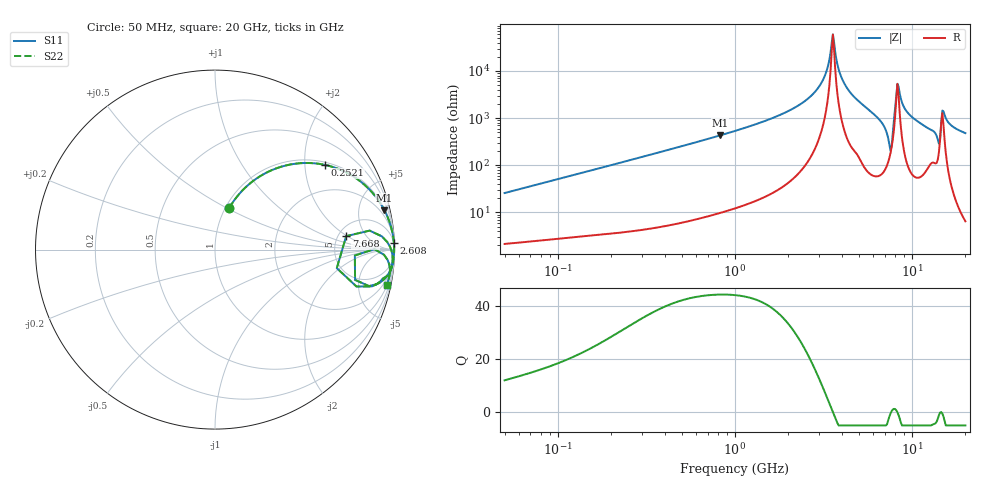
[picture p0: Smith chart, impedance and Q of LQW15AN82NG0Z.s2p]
!Murata Part Number: LQW15AN82NG0Z
!These Parameters are Measured in Series Mode Connection
!  o--[Z]--o
!Port1  Port2
!  o-------o
!Freq. Start=50[MHz] Stop=20[GHz], 401[Steps]
# Hz S RI R 50
!Freq.(Hz) S11(Real) S11(Imag) S21(Real) S21(Imag) S12(Real) S12(Imag) S22(Real) S22(Imag)
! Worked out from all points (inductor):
!   401 points, 50 MHz to 20 GHz, reference 50 ohm
!   read as one part in series: L = 81.5 nH near 51.52 MHz
!   highest Q = 44.2 at 823.1 MHz (marker M1), where L = 83.2 nH
!   self-resonance near 3.572 GHz
!   S11 on the Smith chart (normalised r, x): 50 MHz: 1.04, +0.51; 252.1 MHz: 1.08, +2.54; 2.608 GHz: 4, +53; 7.668 GHz: 5.90, +1.92; 20 GHz: 1.13, -9.63
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5e7  0.0794 0.2318  0.9206 -0.2318  0.9206 -0.2318  0.0794 0.2318
1.364002e8  0.3298 0.4482  0.6702 -0.4482  0.6702 -0.4482  0.3298 0.4482
2.520729e8  0.6138 0.4717  0.3862 -0.4717  0.3862 -0.4717  0.6138 0.4717
3.721004e8  0.7734 0.4059  0.2266 -0.4059  0.2266 -0.4059  0.7734 0.4059
8.230629e8  0.9443 0.2183  0.0557 -0.2183  0.0557 -0.2183  0.9443 0.2183
1e9  0.9625 0.1789  0.0375 -0.1789  0.0375 -0.1789  0.9625 0.1789
1.820564e9  0.9908 0.0825  0.00917 -0.0825  0.00917 -0.0825  0.9908 0.0825
2.608132e9  0.9968 0.0371  0.00317 -0.0371  0.00317 -0.0371  0.9968 0.0371
2.728004e9  0.9972 0.0318  0.00276 -0.0318  0.00276 -0.0318  0.9972 0.0318
3.216634e9  0.9982 0.0124  0.00182 -0.0124  0.00182 -0.0124  0.9982 0.0124
3.572216e9  0.9983 2.62e-05  0.00168 -2.62e-05  0.00168 -2.62e-05  0.9983 2.62e-05
3.908127e9  0.9981 -0.0109  0.00187 0.0109  0.00187 0.0109  0.9981 -0.0109
4.212059e9  0.9977 -0.0203  0.00232 0.0203  0.00232 0.0203  0.9977 -0.0203
6.601595e9  0.9801 -0.1092  0.0199 0.1092  0.0199 0.1092  0.9801 -0.1092
7.442007e9  0.7885 -0.2057  0.2115 0.2057  0.2115 0.2057  0.7885 -0.2057
7.668323e9  0.7311 0.075  0.2689 -0.075  0.2689 -0.075  0.7311 0.075
8.141811e9  0.9743 0.0174  0.0257 -0.0174  0.0257 -0.0174  0.9743 0.0174
8.389408e9  0.9857 -0.0156  0.0143 0.0156  0.0143 0.0156  0.9857 -0.0156
9.600142e9  0.9878 -0.0804  0.0122 0.0804  0.0122 0.0804  0.9878 -0.0804
1.396067e10  0.8582 -0.2035  0.1418 0.2035  0.1418 0.2035  0.8582 -0.2035
1.504638e10  0.9617 -0.0576  0.0383 0.0576  0.0383 0.0576  0.9617 -0.0576
2e10  0.9562 -0.198  0.0438 0.198  0.0438 0.198  0.9562 -0.198
